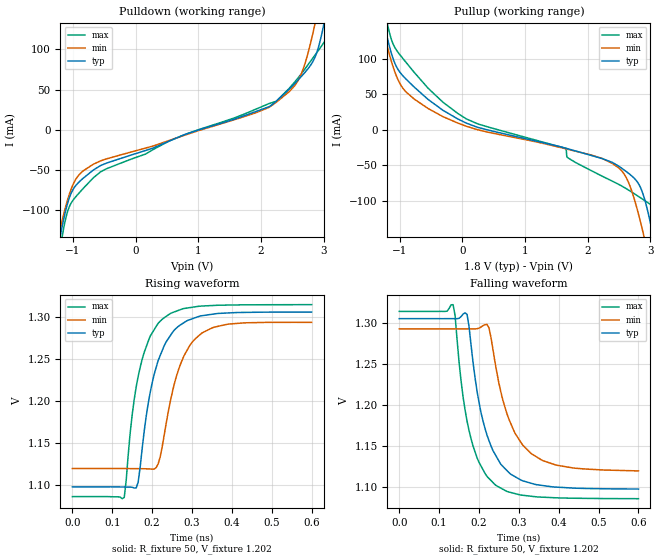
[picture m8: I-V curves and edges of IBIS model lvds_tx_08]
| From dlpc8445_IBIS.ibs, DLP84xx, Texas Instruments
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|   MODEL lvds_tx_08
[Model] lvds_tx_08
Model_type Output
C_comp 1.603p 1.669p 1.519p
Vmeas = 1.2
Vref = 1.2V
Rref = 50
Cref = 0.5pF
[Model Spec]
[Temperature Range]  40 150 -40
[Voltage Range] 1.8 1.62 1.98
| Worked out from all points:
|   slope of the pulldown table from 0 to 0.27 V, typ, clamps not added: 40.2 ohm
|   slope of the pullup table from 0 to 0.27 V, typ, clamps not added: 29.4 ohm
|   rising waveform, R_fixture 50, V_fixture 1.202: 20-80 % time 54.8ps typ, 57.3ps min, 49.3ps max; typ from 1.1 V to 1.3 V
|   falling waveform, R_fixture 50, V_fixture 1.202: 20-80 % time 59ps typ, 67ps min, 51.8ps max; typ from 1.31 V to 1.1 V
[Pulldown]
-1.71V    -379mA     -326.6mA   -450mA
-1.219V   -138.8mA   -128.5mA   -155.2mA
-1.156V   -113.7mA   -107.2mA   -125.3mA
-1.082V   -90.13mA   -85.78mA   -100.4mA
-986.8mV  -72.52mA   -65.87mA   -86.11mA
-675.3mV  -49.89mA   -42.68mA   -59.58mA
2.133V    28.81mA    28.04mA    32.71mA
2.598V    62.26mA    61.76mA    64.94mA
2.861V    89.86mA    131mA      92.56mA
2.993V    126.9mA    180.8mA    107mA
3.125V    182.6mA    234.3mA    129.7mA
3.511V    373.5mA    396.1mA    335mA
[Pullup]
-1.711V   373.5mA    320.4mA    445.7mA
-1.283V   163.6mA    146.1mA    189.8mA
-998.1mV  80.75mA    64.86mA    105.2mA
-549.4mV  42.69mA    29.96mA    58.46mA
62.91mV   9.323mA    4.987mA    15.26mA
1.652V    -25.88mA   -26.67mA   -26.07mA
2.232V    -40.44mA   -40.25mA   -65.14mA
2.607V    -58.08mA   -65.98mA   -82.19mA
2.882V    -90.16mA   -143.9mA   -97.68mA
3.03V     -143.2mA   -201.3mA   -107.4mA
3.172V    -208.9mA   -260.1mA   -145.5mA
3.51V     -379mA     -402.7mA   -338.6mA
[Ramp]
dV/dt_r .125/54.982p .104/57.327p .137/49.496p
dV/dt_f .125/59.135p .104/67.601p .137/51.559p
[Rising Waveform]
R_fixture = 50
V_fixture = 1.202
V_fixture_min = 1.206
V_fixture_max = 1.2
0s        1.098V     1.12V      1.086V
130ps     1.098V     1.12V      1.085V
150ps     1.097V     1.12V      1.184V
165ps     1.104V     1.119V     1.229V
195ps     1.21V      1.119V     1.277V
210ps     1.24V      1.121V     1.288V
225ps     1.259V     1.145V     1.297V
270ps     1.29V      1.242V     1.308V
325ps     1.301V     1.281V     1.312V
600ps     1.305V     1.293V     1.314V
[Falling Waveform]
R_fixture = 50
V_fixture = 1.202
V_fixture_min = 1.206
V_fixture_max = 1.2
0s        1.306V     1.293V     1.314V
135ps     1.306V     1.293V     1.323V
160ps     1.311V     1.293V     1.21V
175ps     1.296V     1.293V     1.169V
195ps     1.217V     1.293V     1.136V
220ps     1.164V     1.299V     1.113V
240ps     1.141V     1.253V     1.103V
275ps     1.118V     1.183V     1.094V
330ps     1.105V     1.142V     1.089V
600ps     1.098V     1.12V      1.086V
